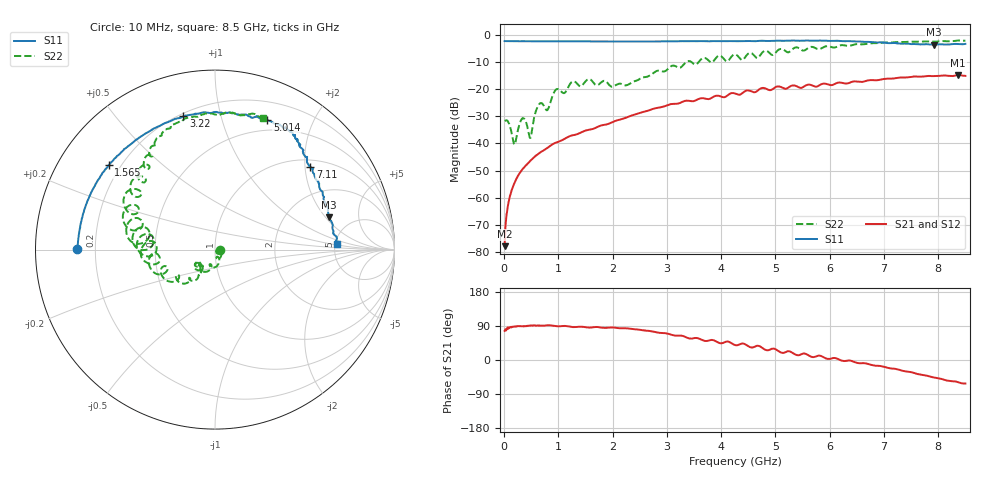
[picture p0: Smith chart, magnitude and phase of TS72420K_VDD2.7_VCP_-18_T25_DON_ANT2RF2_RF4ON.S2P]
!Agilent Technologies,E5071C,MY46417908,A.11.23
!Date: Thu Oct 03 16:41:43 2019
!Data & Calibration Information:
!Freq	S11:SOLT2(ON)	S21:SOLT2(ON)	S12:SOLT2(ON)	S22:SOLT2(ON)
!PortZ  Port1:50+j0  Port2:50+j0
!Above PortZ is port z conversion or system Z0 setting when saving the data.
!When reading, reference impedance value at option line is always used.
# Hz S dB R 50
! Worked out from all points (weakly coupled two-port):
!   1601 points, 10 MHz to 8.5 GHz, reference 50 ohm
!   highest |S21| = -14.78 dB at 8.367 GHz (marker M1); lowest = -77.8 dB at 10 MHz (marker M2)
!   lowest |S11| = -3.6 dB at 7.922 GHz (marker M3), VSWR 4.86, Z = 169 + j108 ohm
!   |S11| at or under -10 dB: nowhere
!   |S22| runs from -40.4 to -2.1 dB; largest |S21 - S12| = 0.0022
!   S11 on the Smith chart (normalised r, x): 10 MHz: 0.13, +0.00; 1.565 GHz: 0.15, +0.34; 3.22 GHz: 0.22, +0.77; 5.014 GHz: 0.38, +1.41; 7.11 GHz: 1.17, +2.14; 8.5 GHz: 5.20, +0.62
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1e7  -2.29 179.8  -77.80 76.8  -76.94 76.1  -31.70 -2.1
8.42875e7  -2.33 177.7  -61.44 83.6  -61.63 84.4  -32.32 -29.5
1.904125e8  -2.35 174.9  -54.67 87.9  -54.59 88.2  -40.40 -25.0
3.177625e8  -2.37 171.6  -50.07 89.1  -50.13 88.9  -31.28 -26.9
3.814375e8  -2.36 170.0  -48.53 89.3  -48.62 89.2  -31.15 -53.2
4.822562e8  -2.37 167.4  -46.43 90.7  -46.49 90.7  -37.99 -40.4
6.520562e8  -2.37 163.1  -43.52 90.6  -43.56 90.7  -25.38 -57.2
7.900188e8  -2.38 159.8  -41.74 91.3  -41.79 91.3  -27.77 -74.4
9.598188e8  -2.38 155.6  -39.63 89.0  -39.67 89.0  -20.08 -90.8
1.426769e9  -2.42 144.8  -35.85 87.8  -35.86 87.5  -18.82 -126.1
1.564731e9  -2.42 141.6  -34.98 85.5  -34.95 85.3  -16.29 -134.8
2.249238e9  -2.47 125.6  -30.47 83.7  -30.43 83.6  -18.60 -129.0
2.843538e9  -2.41 111.8  -26.82 72.1  -26.77 72.1  -13.18 -129.4
3.220281e9  -2.35 103.3  -25.23 64.5  -25.19 64.6  -12.11 -145.4
4.255e9  -2.30 81.7  -21.60 39.5  -21.59 39.6  -7.20 175.8
5.013794e9  -2.17 68.0  -19.12 27.3  -19.10 27.5  -6.30 166.7
5.671769e9  -2.16 58.2  -18.59 8.1  -18.58 8.3  -4.43 138.8
7.088538e9  -3.07 41.7  -16.12 -21.4  -16.17 -21.3  -2.82 111.2
7.109762e9  -3.05 40.9  -16.15 -21.9  -16.17 -22.1  -2.84 110.8
7.921619e9  -3.62 15.9  -15.18 -46.0  -15.09 -46.0  -2.50 88.8
8.367344e9  -3.34 4.8  -14.78 -58.9  -14.85 -58.8  -2.09 74.6
8.5e9  -3.33 2.7  -15.11 -62.1  -15.17 -62.2  -2.16 70.1
